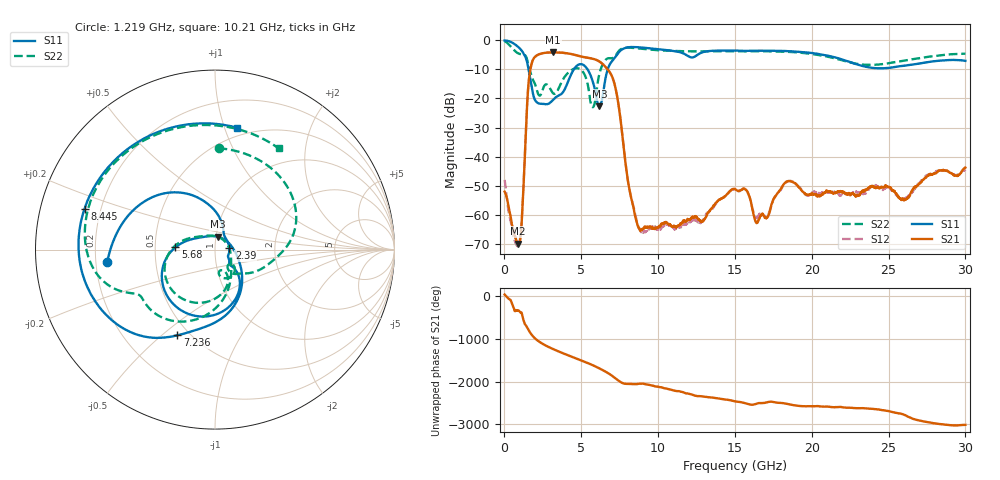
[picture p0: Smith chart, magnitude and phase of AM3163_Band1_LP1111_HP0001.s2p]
!Agilent Technologies,E8364B,MY43040894,A.07.50.67
!Agilent E8364B: A.07.50.67
!Date: Thursday, August 20, 2020 11:57:08
!Correction: S11(Full 2 Port(1,2))
!S21(Full 2 Port(1,2))
!S12(Full 2 Port(1,2))
!S22(Full 2 Port(1,2))
!S2P File: Measurements: S11, S21, S12, S22:
# Hz S  dB  R 50
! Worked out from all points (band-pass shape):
!   3201 points, 10 MHz to 30 GHz, reference 50 ohm
!   highest |S21| = -4.19 dB at 3.178 GHz (marker M1); lowest = -69.7 dB at 891 MHz (marker M2)
!   |S21| within 3 dB of the highest: 1.82 GHz to 6.143 GHz (4.323 GHz wide, 109 % of centre)
!   lowest |S11| = -22.7 dB at 6.177 GHz (marker M3), VSWR 1.16, Z = 51.2 + j7.36 ohm
!   |S11| at or under -10 dB: 1.569 GHz to 4.519 GHz (2.95 GHz wide, 96.9 % of centre); 5.405 GHz to 6.721 GHz (1.316 GHz wide, 21.7 % of centre)
!   |S22| runs from -23.0 to -0.3 dB; largest |S21 - S12| = 0.0051
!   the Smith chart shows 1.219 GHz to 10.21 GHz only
!   S11 on the Smith chart (normalised r, x): 1.219 GHz: 0.25, -0.05; 2.39 GHz: 1.17, +0.02; 5.68 GHz: 0.64, +0.02; 7.236 GHz: 0.43, -0.56; 8.445 GHz: 0.14, +0.15; 10.21 GHz: 0.43, +1.10
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1e7  -0.10 -8.9  -51.94 41.3  -47.89 -52.2  -0.34 -15.6
4.223625e8  -0.64 -55.5  -61.15 -107.5  -62.43 -79.8  -2.25 -92.2
8.909562e8  -2.31 -119.7  -69.73 31.5  -70.41 -46.1  -4.52 167.9
1.218972e9  -4.37 -173.4  -52.51 -179.5  -52.18 159.5  -4.96 88.0
1.650078e9  -12.40 95.2  -11.16 -118.7  -11.16 -118.9  -10.38 -16.7
2.024953e9  -20.84 53.0  -5.54 82.5  -5.55 82.4  -15.65 -53.7
2.390456e9  -21.83 7.1  -4.60 -12.7  -4.61 -12.7  -18.46 -41.8
3.177694e9  -20.38 -35.1  -4.19 -157.8  -4.20 -157.8  -18.27 -78.2
3.946188e9  -16.60 -44.4  -4.40 86.1  -4.42 86.1  -12.38 -79.0
5.014581e9  -8.25 -120.4  -5.64 -65.2  -5.62 -64.9  -10.30 -156.7
5.679984e9  -13.11 176.7  -6.29 -163.1  -6.26 -163.1  -22.65 83.4
6.176694e9  -22.68 76.7  -7.30 112.2  -7.34 112.1  -11.65 -77.1
7.235716e9  -5.65 -113.7  -16.62 -125.0  -16.61 -124.4  -5.22 -154.2
8.444688e9  -2.36 162.6  -58.71 102.1  -58.10 100.7  -2.68 132.8
1.000979e10  -3.11 88.1  -64.15 43.4  -64.83 34.8  -3.45 65.4
1.02066e10  -3.22 79.7  -63.02 27.4  -64.60 26.9  -3.53 57.8
1.5005e10  -3.59 -72.1  -51.03 59.5  -51.37 60.2  -3.78 -92.6
1.642952e10  -3.62 -106.5  -62.69 6.6  -60.89 7.5  -3.79 -127.3
2.000958e10  -4.40 162.3  -52.75 -56.4  -52.43 -52.4  -4.72 135.3
2.27368e10  -7.96 59.9  -52.72 -96.8  -52.43 -95.0  -7.91 20.3
2.500479e10  -9.51 -63.0  -50.32 -167.9  -50.98 -168.3  -7.94 -93.1
3e10  -7.09 103.2  -43.71 -131.5  -44.92 -133.2  -4.63 99.9
